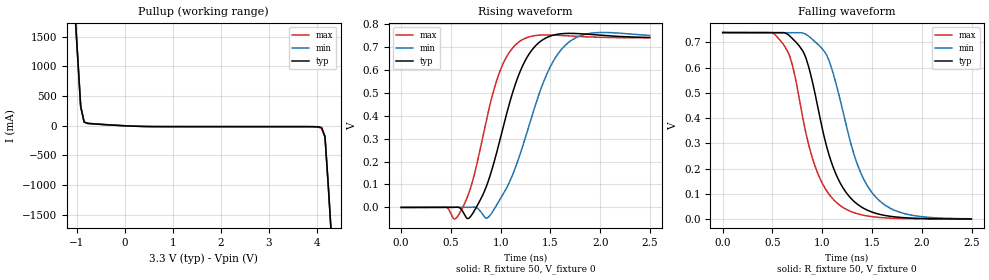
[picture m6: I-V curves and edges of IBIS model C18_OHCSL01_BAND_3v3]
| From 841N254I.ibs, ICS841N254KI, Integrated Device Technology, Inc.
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[Model] C18_OHCSL01_BAND_3v3
Model_type   Open_source
Polarity   Non-Inverting
|   typ   min   max
C_comp   2pF   1.5pF   2.5pF
Vmeas = 0.33V
Rref = 50
Cref = 0
Vref = 0V
|   typ   min   max
[Voltage range]   3.3V   3.135V   3.465V
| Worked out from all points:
|   slope of the pullup table from 0 to 0.495 V, typ, clamps not added: 38 ohm
|   rising waveform, R_fixture 50, V_fixture 0: 20-80 % time 295ps typ, 356ps min, 253ps max; typ from 0 V to 0.74 V
|   falling waveform, R_fixture 50, V_fixture 0: 20-80 % time 302ps typ, 330ps min, 282ps max; typ from 0.738 V to 0 V
[Pullup]
|Voltage   I (typ)   I (min)   I (max)
-3.3V     32.57A     32.54A     32.59A
-1.06V    2.243A     2.239A     2.248A
-987.9mV  1.276A     1.272A     1.28A
-916.2mV  324mA      320.3mA    327.6mA
-844.5mV  62.93mA    59.54mA    66.21mA
-772.8mV  40.5mA     37.42mA    43.47mA
374.8mV   -11.19mA   -10.62mA   -11.67mA
4.104V    -32.38mA   -28.13mA   -39.79mA
4.176V    -185.1mA   -178.9mA   -194.6mA
4.248V    -1.05A     -1.042A    -1.061A
4.32V     -1.996A    -1.987A    -2.009A
6.6V      -32.11A    -32.07A    -32.14A
[Ramp]
|   typ   min   max
dV/dt_r   0.645/0.505n   0.646/0.604n   0.641/0.43n
dV/dt_f   0.59/0.502n   0.589/0.549n   0.59/0.47n
R_load =   50.0000
[Rising Waveform]
R_fixture = 50
V_fixture = 0   | VCC_typ
V_fixture_max = 0   | VCC_max
V_fixture_min = 0   | VCC_min
C_fixture = 0.0p
| Time   typ   min   max
0s        451.1pV    473.2pV    430.3pV
447.9ps   -29.29uV   324.8nV    1.138mV
540.5ps   1.037mV    6.718uV    -50.27mV
693.2ps   -41.84mV   877.5uV    78.5mV
858.4ps   93.67mV    -46.65mV   383.3mV
968.5ps   252.6mV    16.73mV    563.3mV
1.194ns   590mV      230mV      723.8mV
1.449ns   736.7mV    565.8mV    751.2mV
1.657ns   757.8mV    709mV      747.5mV
2.498ns   740mV      748.9mV    738.7mV
[Falling Waveform]
R_fixture = 50
V_fixture = 0   | VCC_typ
V_fixture_max = 0   | VCC_max
V_fixture_min = 0   | VCC_min
C_fixture = 0.0p
| Time   typ   min   max
0s        738.4mV    738.1mV    738.7mV
523ps     738.1mV    738.1mV    730.7mV
668.2ps   726.7mV    737.8mV    650.1mV
765.8ps   687mV      738.2mV    483.8mV
940.9ps   471.3mV    697.6mV    195.2mV
1.059ns   266.8mV    636.7mV    103.7mV
1.176ns   146mV      478.3mV    54.92mV
1.361ns   56.44mV    207.6mV    20.24mV
1.572ns   19.35mV    73.87mV    6.702mV
2.498ns   478.4uV    1.297mV    238.8uV
